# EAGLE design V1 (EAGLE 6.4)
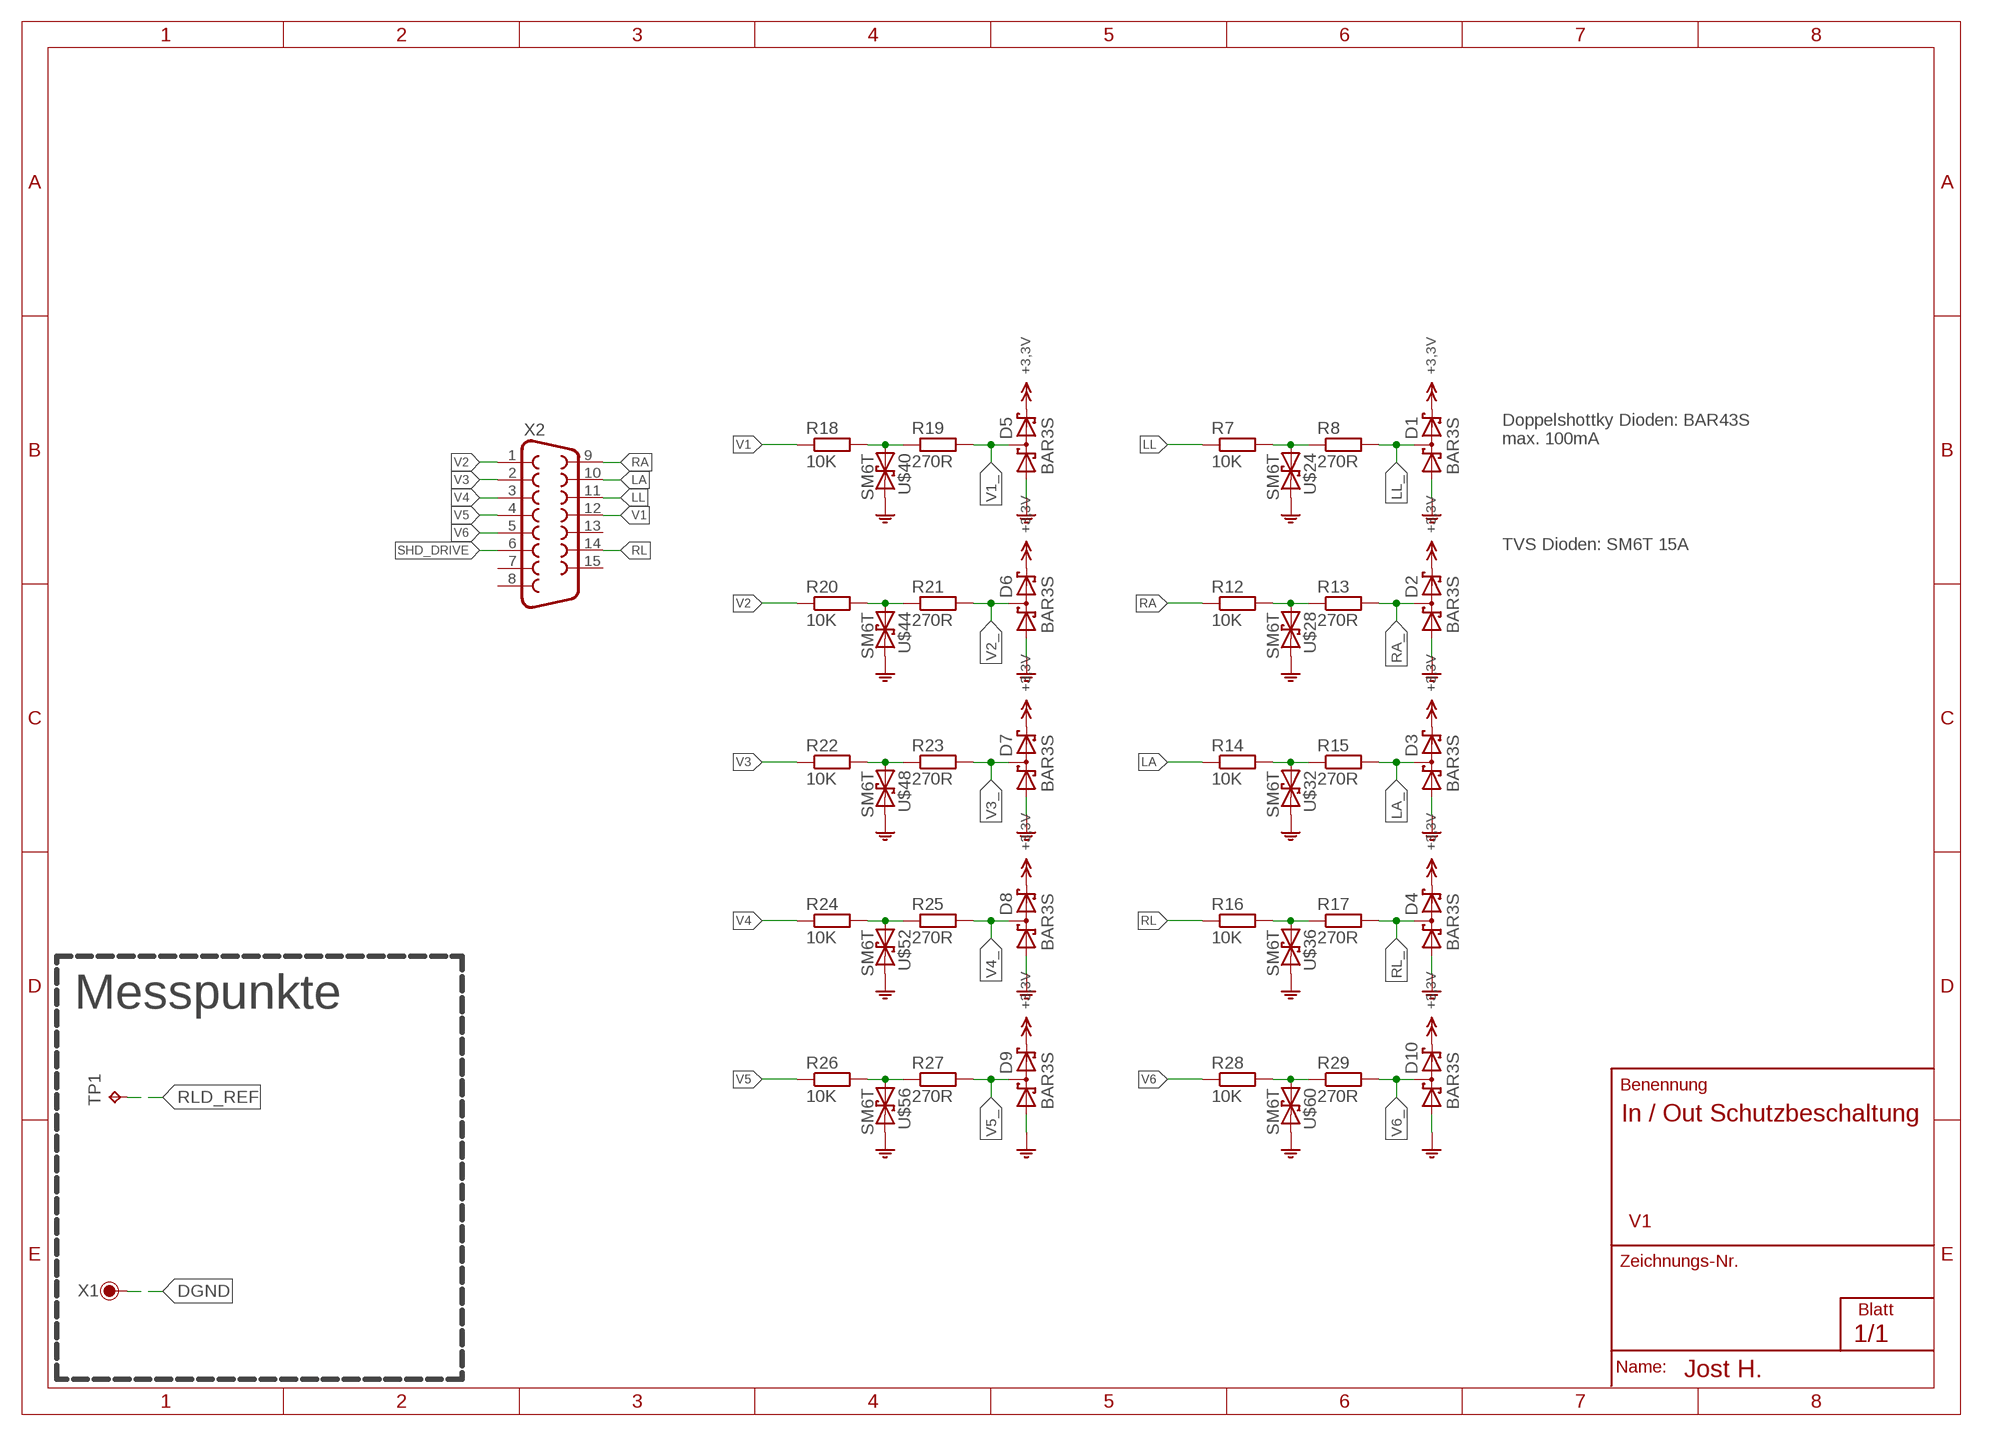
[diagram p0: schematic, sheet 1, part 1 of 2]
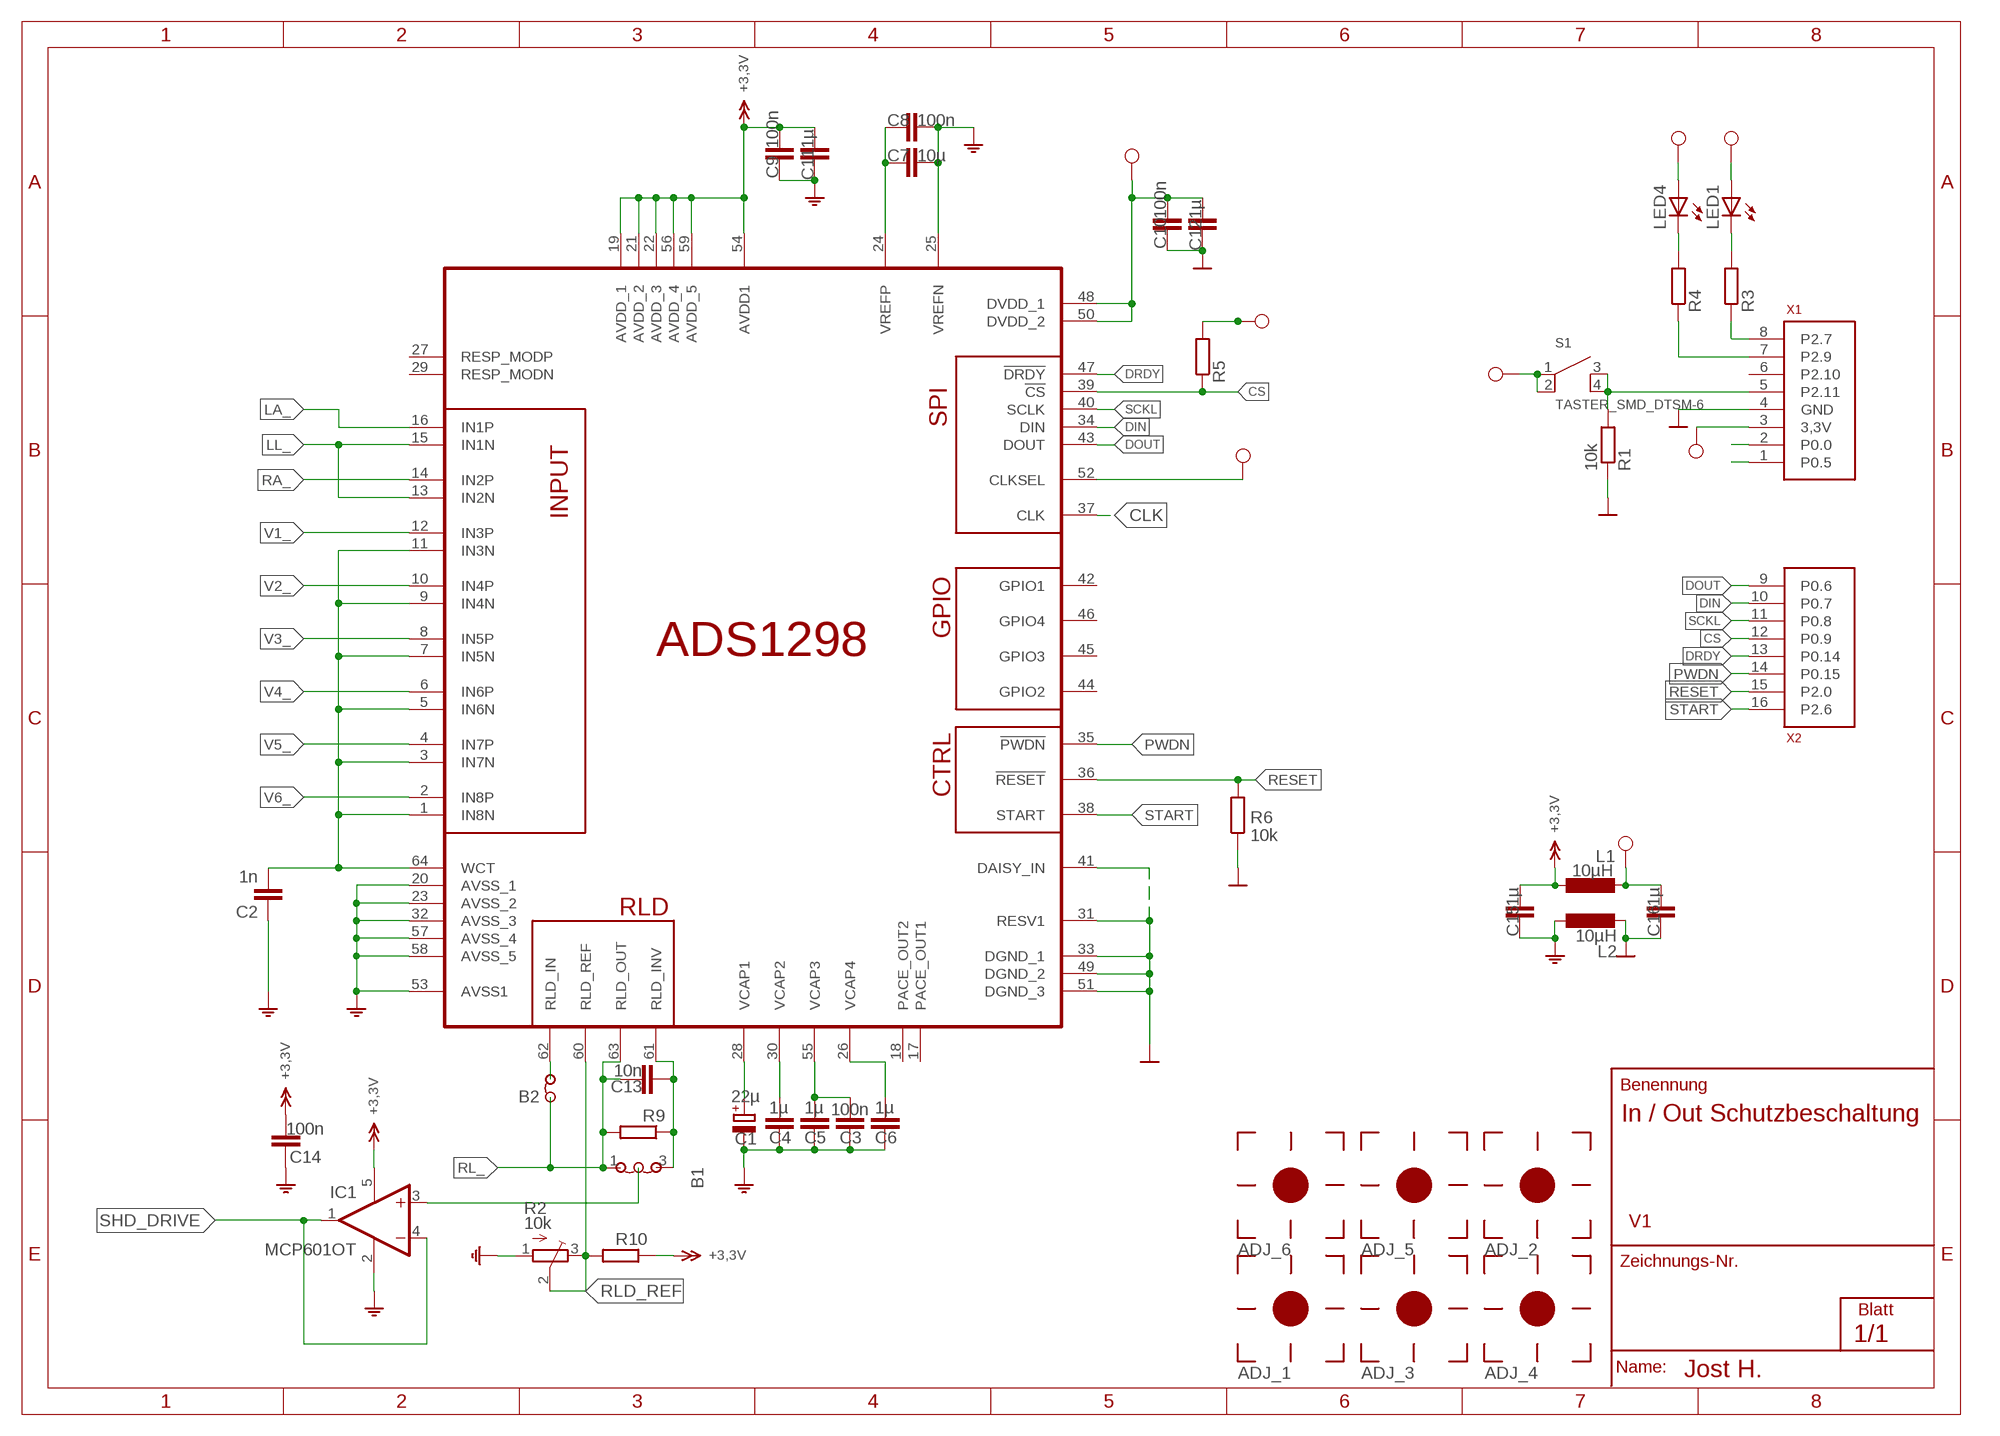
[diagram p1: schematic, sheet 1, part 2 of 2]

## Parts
ADJ_1  FIDUCIAL  [FIDUCIAL]
ADJ_2  FIDUCIAL  [FIDUCIAL]
ADJ_3  FIDUCIAL  [FIDUCIAL]
ADJ_4  FIDUCIAL  [FIDUCIAL]
ADJ_5  FIDUCIAL  [FIDUCIAL]
ADJ_6  FIDUCIAL  [FIDUCIAL]
B1  LÖTBR2  [LÖTBR2NEU]
B2  LÖTBR  [LÖTBR]
C1  22µ  CPOL-EUC/6032-28R  [C/6032-28R]
C2  1n  C-EUC0603K  [C0603K]
C3  100n  C-EUC0603K  [C0603K]
C4  1µ  C-EUC0603K  [C0603K]
C5  1µ  C-EUC0603K  [C0603K]
C6  1µ  C-EUC0603K  [C0603K]
C7  10µ  C-EUC0603K  [C0603K]
C8  100n  C-EUC0603K  [C0603K]
C9  100n  C-EUC0603K  [C0603K]
C10  100n  C-EUC0603K  [C0603K]
C11  1µ  C-EUC0603K  [C0603K]
C12  1µ  C-EUC0603K  [C0603K]
C13  10n  C-EUC0603K  [C0603K]
C14  100n  C-EUC0603K  [C0603K]
C15  1µ  C-EUC0603K  [C0603K]
C16  1µ  C-EUC0603K  [C0603K]
D1  BAR3S  BAS40-04  [SOT23]
D2  BAR3S  BAS40-04  [SOT23]
D3  BAR3S  BAS40-04  [SOT23]
D4  BAR3S  BAS40-04  [SOT23]
D5  BAR3S  BAS40-04  [SOT23]
D6  BAR3S  BAS40-04  [SOT23]
D7  BAR3S  BAS40-04  [SOT23]
D8  BAR3S  BAS40-04  [SOT23]
D9  BAR3S  BAS40-04  [SOT23]
D10  BAR3S  BAS40-04  [SOT23]
IC1  MCP601OT  [SOT23-5]
L1  10µH  L-EU  [1212FPS]
L2  10µH  L-EU  [1212FPS]
LED1  LEDCHIP-LED0603  [CHIP-LED0603]
LED4  LEDCHIP-LED0603  [CHIP-LED0603]
R1  10k  R-EU_R0603  [R0603]
R2  10k  TRIM_EU-3223G  [3223G]
R3  R-EU_R0603  [R0603]
R4  R-EU_R0603  [R0603]
R5  R-EU_R0603  [R0603]
R6  10k  R-EU_R0603  [R0603]
R7  10K  R-EU_R0805  [R0805]
R8  270R  R-EU_R0805  [R0805]
R9  R-EU_R0603  [R0603]
R10  R-EU_R0603  [R0603]
R12  10K  R-EU_R0805  [R0805]
R13  270R  R-EU_R0805  [R0805]
R14  10K  R-EU_R0805  [R0805]
R15  270R  R-EU_R0805  [R0805]
R16  10K  R-EU_R0805  [R0805]
R17  270R  R-EU_R0805  [R0805]
R18  10K  R-EU_R0805  [R0805]
R19  270R  R-EU_R0805  [R0805]
R20  10K  R-EU_R0805  [R0805]
R21  270R  R-EU_R0805  [R0805]
R22  10K  R-EU_R0805  [R0805]
R23  270R  R-EU_R0805  [R0805]
R24  10K  R-EU_R0805  [R0805]
R25  270R  R-EU_R0805  [R0805]
R26  10K  R-EU_R0805  [R0805]
R27  270R  R-EU_R0805  [R0805]
R28  10K  R-EU_R0805  [R0805]
R29  270R  R-EU_R0805  [R0805]
S1  TASTER_SMD_DTSM-6  [TASTER_SMD_DTSM-6]
TP1  TPB1,27  [B1,27]
U$1  ADS1298*PAG*  [TQFP64]
U$2  XMC_2_GO  [XMC_2_GO]
U$24  SM6T  [STPS2L40V]
U$28  SM6T  [STPS2L40V]
U$32  SM6T  [STPS2L40V]
U$36  SM6T  [STPS2L40V]
U$40  SM6T  [STPS2L40V]
U$44  SM6T  [STPS2L40V]
U$48  SM6T  [STPS2L40V]
U$52  SM6T  [STPS2L40V]
U$56  SM6T  [STPS2L40V]
U$60  SM6T  [STPS2L40V]
X1  LÖTPAD  [LÖTPAD]
X2  F15D  [F15D]

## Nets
+3,3V: C9.1 C11.1 C14.1 C15.1 D1.2(C2) D2.2(C2) D3.2(C2) D4.2(C2) D5.2(C2) D6.2(C2) D7.2(C2) D8.2(C2) D9.2(C2) D10.2(C2) IC1.5(V+) L1.P$1 R10.1 U$1.19(AVDD_1) U$1.21(AVDD_2) U$1.22(AVDD_3) U$1.54(AVDD1) U$1.56(AVDD_4) U$1.59(AVDD_5)
AGND: C1.- C2.1 C3.2 C4.2 C5.2 C6.2 C7.1 C8.1 C9.2 C11.2 C14.2 C15.2 D1.1(A1) D2.1(A1) D3.1(A1) D4.1(A1) D5.1(A1) D6.1(A1) D7.1(A1) D8.1(A1) D9.1(A1) D10.1(A1) IC1.2(V-) L2.P$1 R2.1(A) U$1.20(AVSS_1) U$1.23(AVSS_2) U$1.25(VREFN) U$1.32(AVSS_3) U$1.53(AVSS1) U$1.57(AVSS_4) U$1.58(AVSS_5) U$24.K U$28.K U$32.K U$36.K U$40.K U$44.K U$48.K U$52.K U$56.K U$60.K
CLK: U$1.37(CLK)
CS: R5.1 U$1.39(!CS) U$2.12(P0.9)
DGND: C10.2 C12.2 C16.2 L2.P$2 R1.1 R6.1 U$1.31(RESV1) U$1.33(DGND_1) U$1.41(DAISY_IN) U$1.49(DGND_2) U$1.51(DGND_3) U$2.4(GND) X1.1
DIN: U$1.34(DIN) U$2.10(P0.7)
DOUT: U$1.43(DOUT) U$2.9(P0.6)
DRDY: U$1.47(!DRDY) U$2.13(P0.14)
DVDD: C10.1 C12.1 C16.1 L1.P$2 LED1.A LED4.A R5.2 S1.1(1A) S1.2(1B) U$1.48(DVDD_1) U$1.50(DVDD_2) U$1.52(CLKSEL) U$2.3(3,3V)
LA: R14.1 X2.10
LA_: D3.3(C1A2) R15.2 U$1.16(IN1P)
LL: R7.1 X2.11
LL_: D1.3(C1A2) R8.2 U$1.13(IN2N) U$1.15(IN1N)
N$1: U$2.1(P0.5)
N$2: U$2.2(P0.0)
N$3: R4.1 U$2.7(P2.9)
N$4: R3.1 U$2.8(P2.7)
N$5: LED4.C R4.2
N$6: LED1.C R3.2
N$7: C1.+ U$1.28(VCAP1)
N$11: R1.2 S1.3(2A) S1.4(2B) U$2.5(P2.11)
N$12: C4.1 U$1.30(VCAP2)
N$13: C3.1 C5.1 U$1.55(VCAP3)
N$14: C6.1 U$1.26(VCAP4)
N$16: C7.2 C8.2 U$1.24(VREFP)
N$29: B1.3 C13.2 R9.1 U$1.61(RLD_INV)
N$31: B2.1 U$1.62(RLD_IN)
N$37: R7.2 R8.1 U$24.A
N$40: R12.2 R13.1 U$28.A
N$43: R14.2 R15.1 U$32.A
N$46: R16.2 R17.1 U$36.A
N$49: R18.2 R19.1 U$40.A
N$52: R20.2 R21.1 U$44.A
N$55: R22.2 R23.1 U$48.A
N$58: R24.2 R25.1 U$52.A
N$60: R26.2 R27.1 U$56.A
N$62: R28.2 R29.1 U$60.A
PWDN: U$1.35(!PWDN) U$2.14(P0.15)
RA: R12.1 X2.9
RA_: D2.3(C1A2) R13.2 U$1.14(IN2P)
RESET: R6.2 U$1.36(!RESET) U$2.15(P2.0)
RL: R16.1 X2.14
RL_: B1.1 B2.2 C13.1 D4.3(C1A2) R9.2 R17.2 U$1.63(RLD_OUT)
RLD_REF: R2.2(S) R2.3(E) R10.2 TP1.TP U$1.60(RLD_REF)
SCKL: U$1.40(SCLK) U$2.11(P0.8)
SHD_DRIVE: IC1.1(OUT) IC1.4(-IN) X2.6
SHD_DRV_: B1.2 IC1.3(+IN)
START: U$1.38(START) U$2.16(P2.6)
V1: R18.1 X2.12
V1_: D5.3(C1A2) R19.2 U$1.12(IN3P)
V2: R20.1 X2.1
V2_: D6.3(C1A2) R21.2 U$1.10(IN4P)
V3: R22.1 X2.2
V3_: D7.3(C1A2) R23.2 U$1.8(IN5P)
V4: R24.1 X2.3
V4_: D8.3(C1A2) R25.2 U$1.6(IN6P)
V5: R26.1 X2.4
V5_: D9.3(C1A2) R27.2 U$1.4(IN7P)
V6: R28.1 X2.5
V6_: D10.3(C1A2) R29.2 U$1.2(IN8P)
WCT: C2.2 U$1.1(IN8N) U$1.3(IN7N) U$1.5(IN6N) U$1.7(IN5N) U$1.9(IN4N) U$1.11(IN3N) U$1.64(WCT)
Unconnected: U$1.17(PACE_OUT1) U$1.18(PACE_OUT2) U$1.27(RESP_MODP) U$1.29(RESP_MODN) U$1.42(GPIO1) U$1.44(GPIO2) U$1.45(GPIO3) U$1.46(GPIO4) U$2.6(P2.10) X2.7 X2.8 X2.13 X2.15

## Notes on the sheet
- Doppelshottky Dioden: BAR43S
  max. 100mA
- TVS Dioden: SM6T 15A
- Messpunkte

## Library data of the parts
ADJ_1-ADJ_6 = 0_Fiducial:FIDUCIAL
B1 = 3PASSIVE:LÖTBR2
B2 = 3PASSIVE:LÖTBR
C1 = rcl:CPOL-EU: POLARIZED CAPACITOR, European symbol
C2-C16 = rcl:C-EU: CAPACITOR, European symbol
D1-D10 = diode:BAS40-04: Silicon Schottky Diodes General-purpose diode for high-speed switching
IC1 = linear:MCP601: Single Op Amp 2.7V to 6.0V Single Supply CMOS Source: http://ww1.microchip.com/downloads/en/DeviceDoc/21314g.pdf
L1 L2 = 0_Induktivität:L-EU: INDUCTOR, European symbol
LED1 LED4 = led:LED: LED
R1 R3-R10 R12-R29 = rcl:R-EU_: RESISTOR, European symbol
R2 = 0_Poti:TRIM_EU-: POTENTIOMETER
S1 = 1aprojekt:TASTER_SMD_DTSM-6
TP1 = testpad:TP: Test pad
U$1 = burr-brown-5:ADS1298: 8-Channel, 24-Bit Analog-To-Digital Converter With Integrated ECG Front End. Warning: PAG variant (TQFP package) does not have Respiration Module - pins 27 and 29 must stay unconnected! Drawn 23.07.2011 by Tomasz Boleslaw CEDRO (http://www.tomek.cedro.info).
U$2 = 0_XMC Prototyp Board:XMC_2_GO
U$24 U$28 U$32 U$36 U$40 U$44 U$48 U$52 U$56 U$60 = 0_Dioden:SM6T
X1 = 3PASSIVE:LÖTPAD
X2 = con-subd:F15: SUB-D; OC_FARNELL: unknown; OC_NEWARK: unknown

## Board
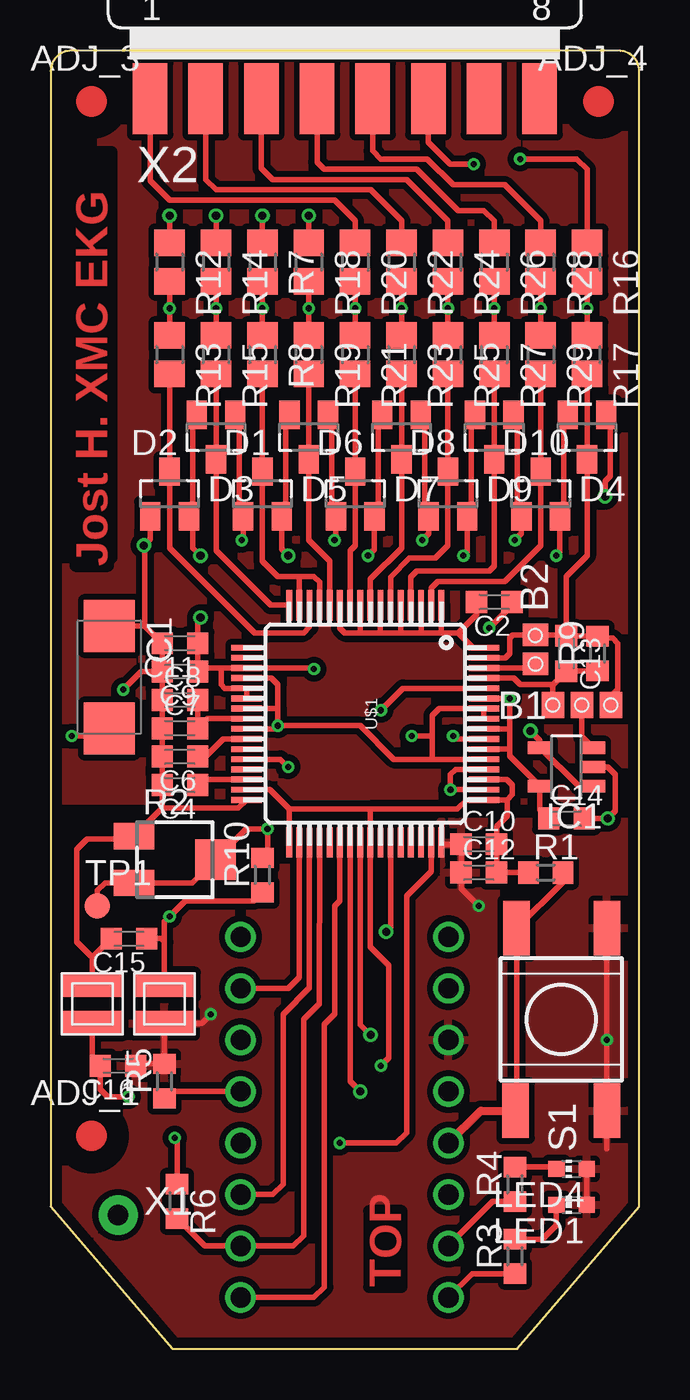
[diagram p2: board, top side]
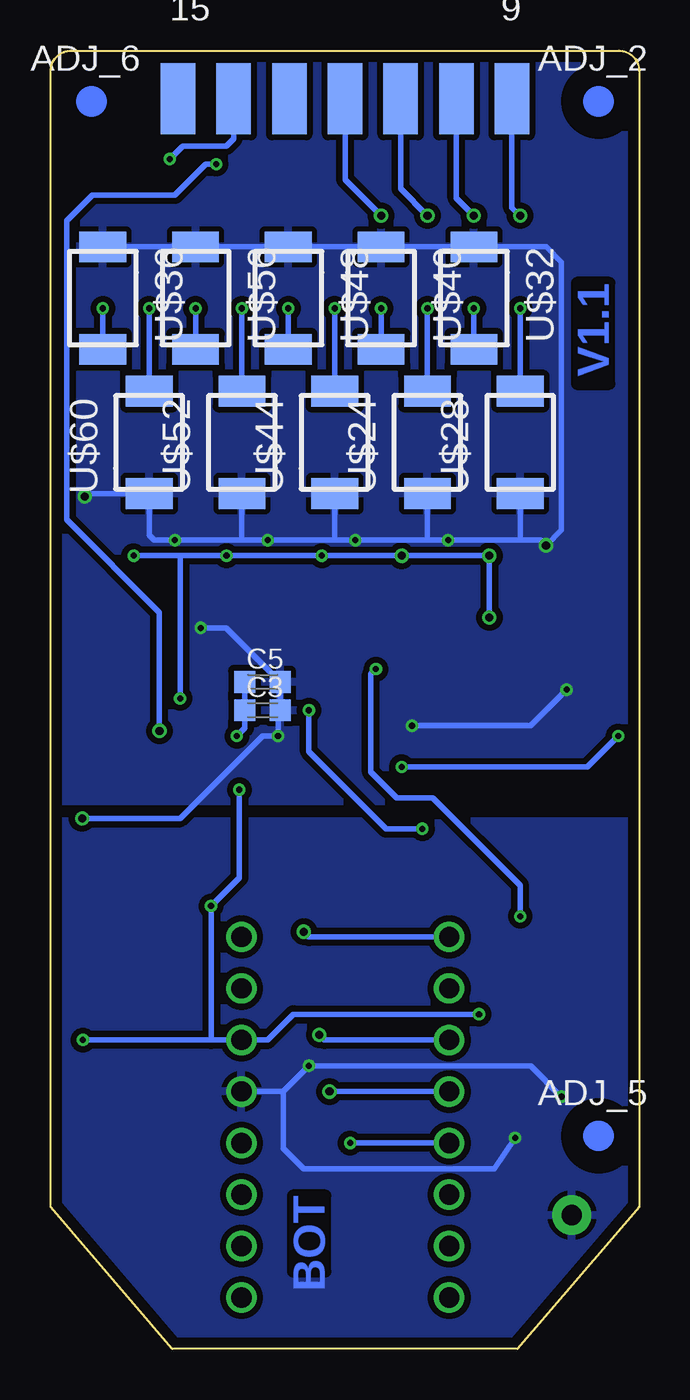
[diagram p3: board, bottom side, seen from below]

Size 29 x 64 mm. Coordinates in mm from the lower left corner, seen from the top.
Outline: 1,64 arc90 0,63 0,7 6,0 23,0 29,7 29,63 arc90 28,64 1,64
Copper layers (1*16): Top 0.035mm / dielectric 1.5mm / Bottom 0.035mm
Design rules "default *": minimum track width 8mil, minimum drill 0.29971875mm, track to track 6mil, track to pad 6mil, pad to pad 6mil, via to via 6mil, smd to smd 6mil, copper to edge 20mil, drill to drill 17mil, minimum pad ring 6mil, minimum via ring 6mil, stop-mask expansion 5mil, vias tented up to drill 0mil, thermal gap 10mil
tRestrict: area 1,39 to 3,59; area 25,62 to 29,64; area 0,62 to 4,64; area 0,59 to 2,60

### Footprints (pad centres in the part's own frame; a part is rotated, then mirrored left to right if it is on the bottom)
LÖTBR2NEU = smd 1.1 x 1.27: 1 -1.429,0; 2 0,0; 3 1.429,0
LÖTBR = smd 1.1 x 1.27: 1 0,0; 2 1.429,0
C/6032-28R = smd 2.55 x 2.5: + 2.525,0; - -2.525,0
C0603K = smd 1.05 x 1.08: 1 -0.875,0; 2 0.875,0
SOT23 = smd 1 x 1.4: 1 -0.95,-1.1; 2 0.95,-1.1; 3 0,1.1
SOT23-5 = smd 0.6 x 1.2: 1 -0.95,-1.306; 2 0,-1.306; 3 0.95,-1.306; 4 0.95,1.306; 5 -0.95,1.306
1212FPS = smd 1.2 x 3: P$1 -0.95,0; P$2 0.95,0
CHIP-LED0603 = smd 0.8 x 0.8: A 0,-0.75; C 0,0.75
R0603 = smd 1 x 1.1: 1 -0.85,0; 2 0.85,0
3223G = smd 2 x 1.3: 1 -2,1.15; 3 -2,-1.15 | smd 2 x 2: 2 2,0
R0805 = smd 1.3 x 1.5: 1 -0.95,0; 2 0.95,0
TASTER_SMD_DTSM-6 = smd 2.7 x 1.3: 1 -4.5,2.25; 2 4.5,2.25; 3 4.5,-2.25; 4 -4.5,-2.2
B1,27 = smd 1.27 x 1.27: TP 0,0
TQFP64 = smd 1.5 x 0.285: 1 -5.85,3.75; 2 -5.85,3.25; 3 -5.85,2.75; 4 -5.85,2.25; 5 -5.85,1.75; 6 -5.85,1.25; 7 -5.85,0.75; 8 -5.85,0.25; 9 -5.85,-0.25; 10 -5.85,-0.75; 11 -5.85,-1.25; 12 -5.85,-1.75; 13 -5.85,-2.25; 14 -5.85,-2.75; 15 -5.85,-3.25; 16 -5.85,-3.75; 33 5.85,-3.75; 34 5.85,-3.25; 35 5.85,-2.75; 36 5.85,-2.25; 37 5.85,-1.75; 38 5.85,-1.25; 39 5.85,-0.75; 40 5.85,-0.25; 41 5.85,0.25; 42 5.85,0.75; 43 5.85,1.25; 44 5.85,1.75; 45 5.85,2.25; 46 5.85,2.75; 47 5.85,3.25; 48 5.85,3.75 | smd 0.285 x 1.5: 17 -3.75,-5.85; 18 -3.25,-5.85; 19 -2.75,-5.85; 20 -2.25,-5.85; 21 -1.75,-5.85; 22 -1.25,-5.85; 23 -0.75,-5.85; 24 -0.25,-5.85; 25 0.25,-5.85; 26 0.75,-5.85; 27 1.25,-5.85; 28 1.75,-5.85; 29 2.25,-5.85; 30 2.75,-5.85; 31 3.25,-5.85; 32 3.75,-5.85; 49 3.75,5.85; 50 3.25,5.85; 51 2.75,5.85; 52 2.25,5.85; 53 1.75,5.85; 54 1.25,5.85; 55 0.75,5.85; 56 0.25,5.85; 57 -0.25,5.85; 58 -0.75,5.85; 59 -1.25,5.85; 60 -1.75,5.85; 61 -2.25,5.85; 62 -2.75,5.85; 63 -3.25,5.85; 64 -3.75,5.85
XMC_2_GO = drill 1: 1 1.88,-37.34; 2 1.88,-34.8; 3 1.88,-32.26; 4 1.88,-29.72; 5 1.88,-27.18; 6 1.88,-24.64; 7 1.88,-22.1; 8 1.88,-19.56; 9 12.12,-37.34; 10 12.12,-34.8; 11 12.12,-32.26; 12 12.12,-29.72; 13 12.12,-27.18; 14 12.12,-24.64; 15 12.12,-22.1; 16 12.12,-19.56
STPS2L40V = smd 1.52 x 2.3: A 2.525,0; K -2.525,0
LÖTPAD = drill 1 pad 1.93: 1 0,0
F15D = smd 1.7 x 3.5: 1 -9.601,-6.045; 2 -6.858,-6.045; 3 -4.115,-6.045; 4 -1.372,-6.045; 5 1.372,-6.045; 6 4.115,-6.045; 7 6.858,-6.045; 8 9.601,-6.045 | smd 1.7 x 3.5 bottom: 9 -8.23,-6.045; 10 -5.486,-6.045; 11 -2.743,-6.045; 12 0,-6.045; 13 2.743,-6.045; 14 5.486,-6.045; 15 8.23,-6.045

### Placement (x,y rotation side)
ADJ_1  2,10.5 0 top
ADJ_2  2,61.5 0 bottom
ADJ_3  2,61.5 0 top
ADJ_4  27,61.5 0 top
ADJ_5  2,10.5 0 bottom
ADJ_6  27,61.5 0 bottom
B1  26.18,31.74 180 top
B2  23.89,33.77 90 top
C1  2.88,33.11 270 top
C2  21.86,36.82 180 top
C3  18.56,31.48 0 bottom
C4  6.37,27.8 180 top
C5  18.56,32.88 0 bottom
C6  6.37,29.2 180 top
C7  6.37,30.59 0 top
C8  6.37,31.99 0 top
C9  6.37,33.39 180 top
C10  21.1,24.88 0 top
C11  6.37,34.78 180 top
C12  21.1,23.48 0 top
C13  25.42,34.28 270 top
C14  25.42,26.15 0 top
C15  3.86,20.22 180 top
C16  3.32,13.96 180 top
D1  10.43,42.15 0 top
D2  5.86,42.15 0 top
D3  8.15,44.94 180 top
D4  26.43,44.94 180 top
D5  12.72,44.94 180 top
D6  15,42.15 0 top
D7  17.29,44.94 180 top
D8  19.58,42.15 0 top
D9  21.86,44.94 180 top
D10  24.15,42.15 0 top
IC1  25.42,28.69 90 top
L1  5.61,17 270 top
L2  2.05,17 270 top
LED1  25.67,7.1 90 top
LED4  25.67,8.88 90 top
R1  24.4,23.48 0 top
R2  6.11,24.12 0 top
R3  22.88,4.56 90 top
R4  22.88,8.11 90 top
R5  5.61,13.19 90 top
R6  6.23,7.27 270 top
R7  10.43,53.58 270 top
R8  10.43,49.01 270 top
R9  26.94,34.28 90 top
R10  10.43,23.35 90 top
R12  5.86,53.58 270 top
R13  5.86,49.01 270 top
R14  8.15,53.58 270 top
R15  8.15,49.01 270 top
R16  26.43,53.58 270 top
R17  26.43,49.01 270 top
R18  12.72,53.58 270 top
R19  12.72,49.01 270 top
R20  15,53.58 270 top
R21  15,49.01 270 top
R22  17.29,53.58 270 top
R23  17.29,49.01 270 top
R24  19.58,53.58 270 top
R25  19.58,49.01 270 top
R26  21.86,53.58 270 top
R27  21.86,49.01 270 top
R28  24.15,53.58 270 top
R29  24.15,49.01 270 top
S1  25.16,16.24 270 top
TP1  2.3,21.83 0 top
U$1  15.5,30.82 270 top
U$2  21.48,-17.03 180 top
U$24  10.43,44.69 90 bottom
U$28  5.86,44.69 90 bottom
U$32  8.15,51.8 270 bottom
U$36  26.43,51.8 270 bottom
U$40  12.72,51.8 270 bottom
U$44  15,44.69 90 bottom
U$48  17.29,51.8 270 bottom
U$52  19.58,44.69 90 bottom
U$56  21.86,51.8 270 bottom
U$60  24.15,44.69 90 bottom
X1  3.32,6.59 0 top
X2  14.5,67.68 0 top

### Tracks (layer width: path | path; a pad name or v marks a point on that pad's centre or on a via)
3,3V
  pour Top (isolate 0.3): 0,64 29,64 29,27 0,27
+3,3V  (via drill 0.3, 0.4)
  Top 0.28: 11.57,45.71 11.77,45.71 D5.2 11.77,45.96 11.57,45.96 11.57,41.05 D1.2 11.38,39.42 v11.7,39.1 | D7.2 16.34,45.96 16.15,45.96 16.15,41.05 D6.2 15.95,39.42 v15.64,39.1 | D9.2 20.91,46.09 20.85,46.09 20.85,45.96 20.72,45.96 20.72,41.05 D8.2 20.53,39.29 v20.34,39.1 | D4.2 25.48,45.96 25.29,45.96 25.29,41.05 D10.2 25.1,39.29 v24.91,39.1 | 8.4,33.56 U$1.19 12.92,33.56 v12.97,33.51 | 8.4,33.56 7.42,33.56 C9.1 C11.1 7.24,35.91 v7.38,36.05 | U$1.22 U$1.21 8.59,32.56 8.4,32.75 8.4,33.56 | 7,41.05 7,39.48 v7.38,39.1 | D3.2 7,46.04 7,41.05 | 7,41.05 D2.2 | C14.1 24.11,26.58 IC1.5 22.62,29.23 22.62,29.56 | U$1.54 22.62,29.56 | 22.62,30.56 U$1.56 | 22.62,30.56 22.62,29.56 | U$1.59 v22.62,32.06 22.62,30.56 | L1.P$1 5.61,20.05 | 5.61,20.05 5.61,21.07 v5.86,21.32 6.62,22.08 10.01,22.08 R10.1 | C15.1 5.44,20.22 5.61,20.05
  Bottom 0.28: v20.34,39.1 v15.64,39.1 v11.7,39.1 v7.38,39.1 v7.38,36.05 | v20.34,39.1 v24.91,39.1 | v20.34,39.1 22.62,39.1 v22.62,32.06 | v5.86,21.32 5.86,22.85 10.18,27.16 11.96,27.16 13.23,28.43 13.23,33.26 v12.97,33.51
AGND  (via drill 0.3, 0.4)
  Top 0.28: D3.1 9.1,45.96 9.29,45.96 9.29,41.05 D1.1 9.48,39.93 v9.42,39.86 | D5.1 13.67,45.71 13.86,45.71 13.86,41.05 D6.1 14.05,39.93 v13.99,39.86 | D9.1 22.81,45.96 23.01,45.96 23.01,41.05 D10.1 23.2,40.18 v22.88,39.86 | 18.56,45.72 D7.1 18.24,45.71 18.43,45.71 18.43,41.05 D8.1 18.63,40.18 v18.31,39.86 | C9.2 C8.1 C7.1 C6.2 C4.2 5.49,26.66 | C9.2 C11.2 4.64,35.64 | C1.- 4.64,35.64 | v11.19,30.72 11.19,31.56 | 11.19,31.56 11.19,32.75 10.88,33.06 U$1.20 | U$1.23 11.19,31.56 | v3.57,32.5 4.46,33.39 C9.2 | U$1.57 U$1.58 19.15,31.56 18.81,31.23 18.81,30.21 | D2.1 4.91,39.93 v4.59,39.61 4.64,39.56 4.64,35.64 | D4.1 27.58,45.85 27.58,43.04 27.32,42.78 v27.32,42.02 | C14.2 v27.45,26.15 27.83,26.53 27.83,27.93 27.83,28.31 27.45,28.69 IC1.2 | v11.19,30.72 15.26,30.72 16.91,29.06 18.81,29.06 | v11.19,30.72 11.04,30.56 U$1.25 | 5.49,26.66 9.24,26.66 U$1.32 | 18.81,29.06 U$1.53 | 18.81,30.21 18.81,29.06 | v17.8,30.21 18.81,30.21 | 5.49,26.66 R2.1 3.98,25.13 1.8,25.13 1.29,24.62 1.29,20.05 2.05,19.29 | C2.1 22.74,36.67 v21.61,35.55 | L2.P$1 2.05,19.29 | 2.05,19.29 C15.2
  Bottom 0.28: 5.86,39.86 4.84,39.86 v4.59,39.61 3.83,40.37 3.83,53.58 4.57,54.33 U$36.K U$56.K U$48.K U$40.K U$32.K | 5.86,39.86 v9.42,39.86 10.43,39.86 | 10.43,39.86 v13.99,39.86 15,39.86 | 15,39.86 v18.31,39.86 19.58,39.86 | 19.58,39.86 v22.88,39.86 23.89,39.86 24.15,40.12 U$60.K 27.18,42.16 v27.32,42.02 | v11.19,30.72 5.35,30.72 v3.57,32.5 | U$24.K 10.43,39.86 | U$44.K 15,39.86 | U$52.K 19.58,39.86 | v27.45,26.15 22.62,26.15 18.56,30.21 v17.8,30.21 17.8,31.37 C3.2 C5.2 20.35,35.55 v21.61,35.55 | U$28.K 5.86,39.86
  pour Bottom (isolate 0.3): -1,27 -1,65 30,65 30,27
CS  (via drill 0.4)
  Top 0.28: U$1.39 14.75,13.19 v15.26,12.69 | U$2.12 5.95,12.69 R5.1
  Bottom 0.28: U$2.12 v15.26,12.69
DGND  (via drill 0.3)
  Top 0.28: U$1.33 11.75,26.61 | 11.75,26.61 10.79,27.56 U$1.31 | 22.5,27.06 U$1.49 20.49,27.06 20.03,26.61 15.75,26.61 | U$1.51 22.48,28.06 22.75,27.8 22.75,27.32 22.5,27.06 | 22.5,27.06 22.5,26.27 21.98,25.75 C10.2 C12.2 R1.1 | v16.27,13.96 16.66,14.34 16.66,18.91 15.75,19.81 U$1.41 15.75,26.61 | 11.75,26.61 15.75,26.61 | R6.1 6.23,10.26 v6.11,10.4 | L2.P$2 2.05,14.35 C16.2 2.45,12.8 2.81,12.43 v3.83,12.43
  Bottom 0.28: U$2.4 17.54,12.69 | 17.54,12.69 v16.27,13.96 5.35,13.96 v3.83,12.43 | v6.11,10.4 7.13,8.88 16.53,8.88 17.54,9.89 17.54,12.69
  pour Bottom (isolate 0.3): 0,26 29,26 29,0 0,0
DIN
  Top 0.28: U$2.10 11.7,17.77 12.25,18.31 U$1.34
DOUT  (via drill 0.4)
  Top 0.28: v16.53,20.56 16.75,20.78 U$1.43
  Bottom 0.28: U$2.9 16.27,20.31 v16.53,20.56
DRDY  (via drill 0.3)
  Top 0.28: U$1.47 18.75,23.55 17.54,22.34 17.54,10.65 17.04,10.15 v14.24,10.15
  Bottom 0.28: v14.24,10.15 U$2.13
DVDD  (via drill 0.3)
  Top 0.28: U$1.48 19.25,24.88 C10.1 C12.1 20.23,22.7 v21.1,21.83 | 27.41,9.87 S1.2 v27.41,15.23 S1.1 | LED1.A LED4.A | U$1.52 19.96,28.56 19.7,28.31 v19.7,27.56 U$1.50 | v7.89,16.5 7.45,16.05 L1.P$2 R5.2 4.28,14.04 C16.1
  Bottom 0.28: 21.1,15.23 U$2.3 18.3,15.23 17.04,16.5 v7.89,16.5 | 21.1,15.23 v27.41,15.23 | 21.1,15.23 v21.1,21.83 19.7,23.23 v19.7,27.56
  pour Top (isolate 0.3): -1,26 30,26 30,-1 -1,-1
LA  (via drill 0.4)
  Top 0.28: R14.1 v8.15,55.87
  Bottom 0.28: v8.15,55.87 9.01,56.73 X2.10
LA_
  Top 0.28: R15.2 D3.3 8.15,39.36 10.84,36.66 U$1.16
LL  (via drill 0.4)
  Top 0.28: R7.1 v10.43,55.87
  Bottom 0.28: v10.43,55.87 11.75,57.19 X2.11
LL_
  Top 0.28: R8.2 D1.3 10.43,38.85 11.19,38.09 12.25,38.09 | 12.25,38.09 12.97,38.09 13.25,37.81 U$1.13 | U$1.15 12.25,38.09
N$3
  Top 0.28: U$2.7 21.8,7.26 R4.1
N$4
  Top 0.28: U$2.8 20.78,3.71 R3.1
N$5
  Top 0.28: LED4.C 24.83,8.96 R4.2
N$6
  Top 0.28: LED1.C 24.92,6.09 24.24,5.41 R3.2
N$7  (via drill 0.3)
  Top 0.28: U$1.28 11.32,29.06 v11.7,28.69 | v1.03,30.21 2.51,30.21 C1.+
  Bottom 0.28: v11.7,28.69 2.56,28.69 v1.03,30.21
N$11
  Top 0.28: S1.3 22.96,11.79 S1.4 25.25,23.03 R1.2
  Top 0.406: U$2.5 21.2,11.74 S1.3
N$12
  Top 0.28: C4.1 7.51,28.06 U$1.30
N$13  (via drill 0.3)
  Top 0.28: U$1.55 19.98,30.06 v19.83,30.21
  Bottom 0.28: v19.83,30.21 19.44,30.61 C3.1 C5.1
N$14
  Top 0.28: U$1.26 8.51,30.06 7.64,29.2 C6.1
N$16
  Top 0.28: C8.2 C7.2 7.71,31.06 U$1.24
N$29
  Top 0.28: R9.1 25.44,33.43 C13.2 24.77,32.75 24.66,32.75 | U$1.61 22.82,33.06 23.13,32.75 24.66,32.75 | B1.3 24.75,32.66 24.66,32.75
N$31
  Top 0.28: U$1.62 23.69,33.56 B2.1
N$37  (via drill 0.3)
  Top 0.28: R8.1 v10.43,51.29 R7.2
  Bottom 0.28: v10.43,51.29 U$24.A
N$40  (via drill 0.3)
  Top 0.28: R13.1 v5.86,51.29 R12.2
  Bottom 0.28: v5.86,51.29 U$28.A
N$43  (via drill 0.3)
  Top 0.28: R15.1 v8.15,51.29 R14.2
  Bottom 0.28: U$32.A v8.15,51.29
N$46  (via drill 0.3)
  Top 0.28: R17.1 v26.43,51.29 R16.2
  Bottom 0.28: v26.43,51.29 U$36.A
N$49  (via drill 0.3)
  Top 0.28: R19.1 v12.72,51.29 R18.2
  Bottom 0.28: U$40.A v12.72,51.29
N$52  (via drill 0.3)
  Top 0.28: R21.1 v15,51.29 R20.2
  Bottom 0.28: v15,51.29 U$44.A
N$55  (via drill 0.3)
  Top 0.28: R23.1 v17.29,51.29 R22.2
  Bottom 0.28: U$48.A v17.29,51.29
N$58  (via drill 0.3)
  Top 0.28: R25.1 v19.58,51.29 R24.2
  Bottom 0.28: v19.58,51.29 U$52.A
N$60  (via drill 0.3)
  Top 0.28: R27.1 v21.86,51.29 R26.2
  Bottom 0.28: U$56.A v21.86,51.29
N$62  (via drill 0.3)
  Top 0.28: R29.1 v24.15,51.29 R28.2
  Bottom 0.28: v24.15,51.29 U$60.A
PWDN
  Top 0.28: U$2.14 10.94,7.61 11.45,8.11 11.45,16.5 12.75,17.8 U$1.35
RA  (via drill 0.4)
  Top 0.28: R12.1 v5.86,55.87
  Bottom 0.28: v5.86,55.87 6.27,56.27 X2.9
RA_
  Top 0.28: R13.2 D2.3 5.86,39.48 10.05,35.29 12.46,35.29 12.75,35.58 U$1.14
RESET
  Top 0.28: U$1.36 13.23,17 12.46,16.24 12.46,5.57 11.96,5.07 U$2.15 7.58,5.07 R6.2
RL  (via drill 0.3)
  Top 0.28: R16.1 26.43,58.15 25.93,58.66 v23.13,58.66
  Bottom 0.28: X2.14 19.98,59.65 20.34,59.3 22.5,59.3 v23.13,58.66
RL_
  Top 0.28: R17.2 D4.3 26.43,39.1 25.42,38.09 C13.1 | U$1.63 22.41,34.06 22.62,34.28 22.62,35.04 22.78,35.2 B2.2 25.37,35.2 C13.1 | C13.1 26.92,35.15 R9.2 27.03,35.04 27.7,35.04 27.96,34.78 27.96,32.5 27.61,32.15 B1.1
RLD_REF  (via drill 0.3)
  Top 0.28: v16.27,31.48 17.36,32.56 U$1.60 | R10.2 10.69,24.46 v10.69,25.64 9.64,25.64 R2.2 6.96,22.97 R2.3 2.68,22.97 2.3,22.59 TP1.TP
  Bottom 0.28: v10.69,25.64 12.46,25.64 16.27,29.45 v16.27,31.48
SCKL  (via drill 0.4)
  Top 0.28: v15.77,15.48 15.25,15.98 U$1.40
  Bottom 0.28: U$2.11 15.51,15.23 v15.77,15.48
SHD_DRIVE  (via drill 0.3, 0.4)
  Top 0.28: X2.6 18.61,59.5 19.7,58.41 v20.85,58.41 | IC1.1 26.01,27.74 IC1.4 24.11,29.99 v23.64,30.47
  Bottom 0.28: v23.64,30.47 23.64,36.31 28.21,40.88 28.21,55.61 26.94,56.88 22.88,56.88 21.35,58.41 v20.85,58.41
SHD_DRV_
  Top 0.28: B1.2 26.18,30.18 IC1.3
START
  Top 0.28: U$2.16 12.97,2.53 13.49,3.04 13.48,15.99 14,16.5 13.99,21.83 14.25,22.09 U$1.38
V1  (via drill 0.4)
  Top 0.28: R18.1 v12.72,55.87
  Bottom 0.28: v12.72,55.87 14.5,57.64 X2.12
V1_
  Top 0.28: R19.2 D5.3 12.72,39.86 13.75,38.83 U$1.12
V2
  Top 0.28: R20.1 15,55.61 13.99,56.63 5.86,56.63 4.89,57.59 X2.1
V2_
  Top 0.28: R21.2 D6.3 15,39.61 14.75,39.36 U$1.10
V3
  Top 0.28: R22.1 17.29,55.61 15.77,57.14 8.15,57.14 7.64,57.64 X2.2
V3_
  Top 0.28: R23.2 D7.3 17.29,39.48 15.75,37.94 U$1.8
V4
  Top 0.28: R24.1 19.58,55.61 17.54,57.64 10.94,57.64 10.38,58.2 X2.3
V4_
  Top 0.28: R25.2 D8.3 19.58,39.61 18.94,38.98 17.67,38.98 16.75,38.05 U$1.6
V5
  Top 0.28: R26.1 21.86,55.61 21.35,56.12 20.08,56.12 18.05,58.15 13.48,58.15 13.12,58.51 X2.4
V5_
  Top 0.28: R27.2 D9.3 21.86,38.59 21.61,38.34 18.05,38.34 17.75,38.04 U$1.4
V6
  Top 0.28: R28.1 24.15,55.61 22.37,57.39 19.83,57.39 18.56,58.66 16.27,58.66 15.87,59.07 X2.5
V6_
  Top 0.28: R29.2 D10.3 24.15,39.61 22.37,37.83 19.07,37.83 18.75,37.52 U$1.2
WCT
  Top 0.28: U$1.11 14.25,35.54 14.5,35.29 15.25,35.29 | 15.25,35.29 16.27,35.29 | 16.27,35.29 17.25,35.29 | 17.25,35.29 18.25,35.29 | 18.25,35.29 19.25,35.29 | U$1.7 16.25,35.31 16.27,35.29 | U$1.9 15.25,35.29 | U$1.5 17.25,35.29 | U$1.3 18.25,35.29 | U$1.1 19.25,35.29 | 19.25,35.29 20.08,35.29 | 20.08,35.29 20.81,34.56 U$1.64 | C2.2 20.99,36.2 20.08,35.29

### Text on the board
Top: Jost H. XMC EKG | TOP
Bottom: V1.1 | BOT
tDocu: ANALOG / PLANE | DIGITAL / PLANE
